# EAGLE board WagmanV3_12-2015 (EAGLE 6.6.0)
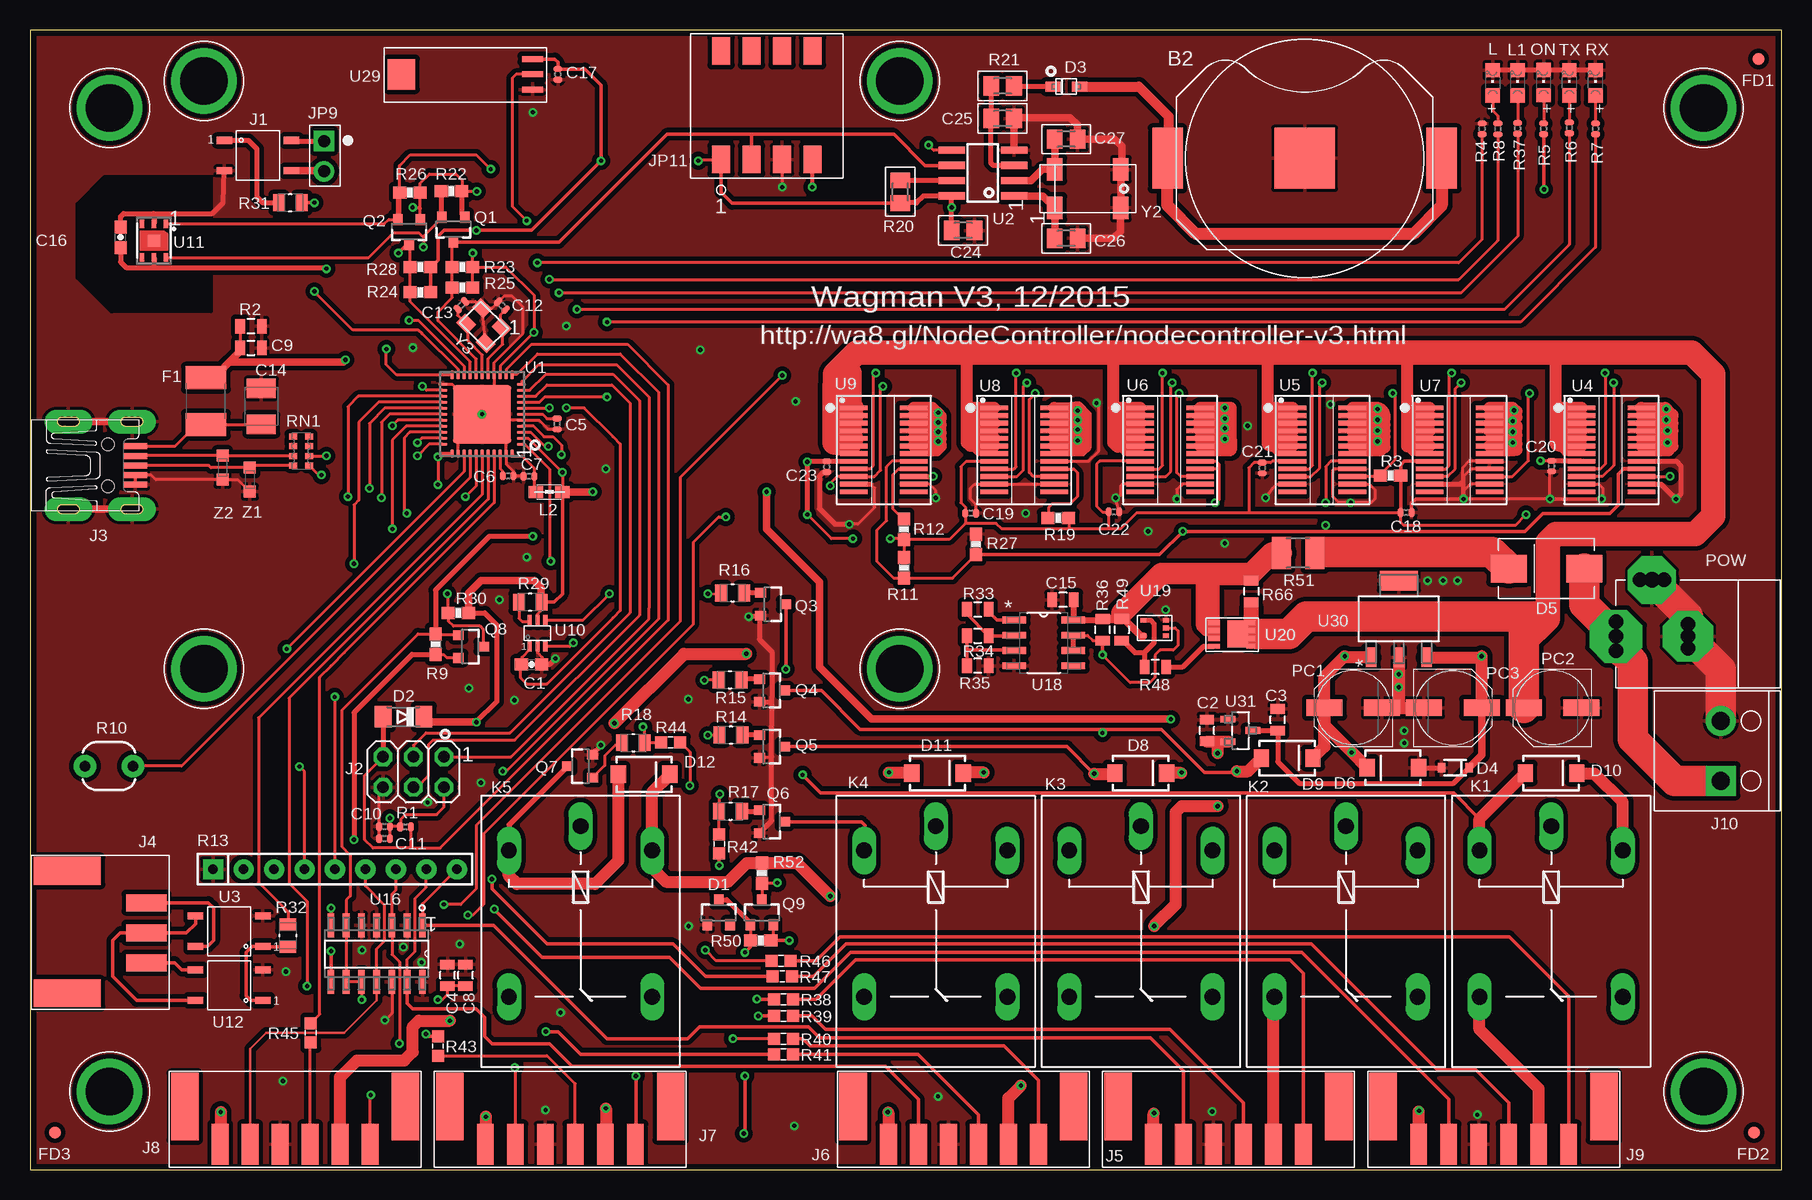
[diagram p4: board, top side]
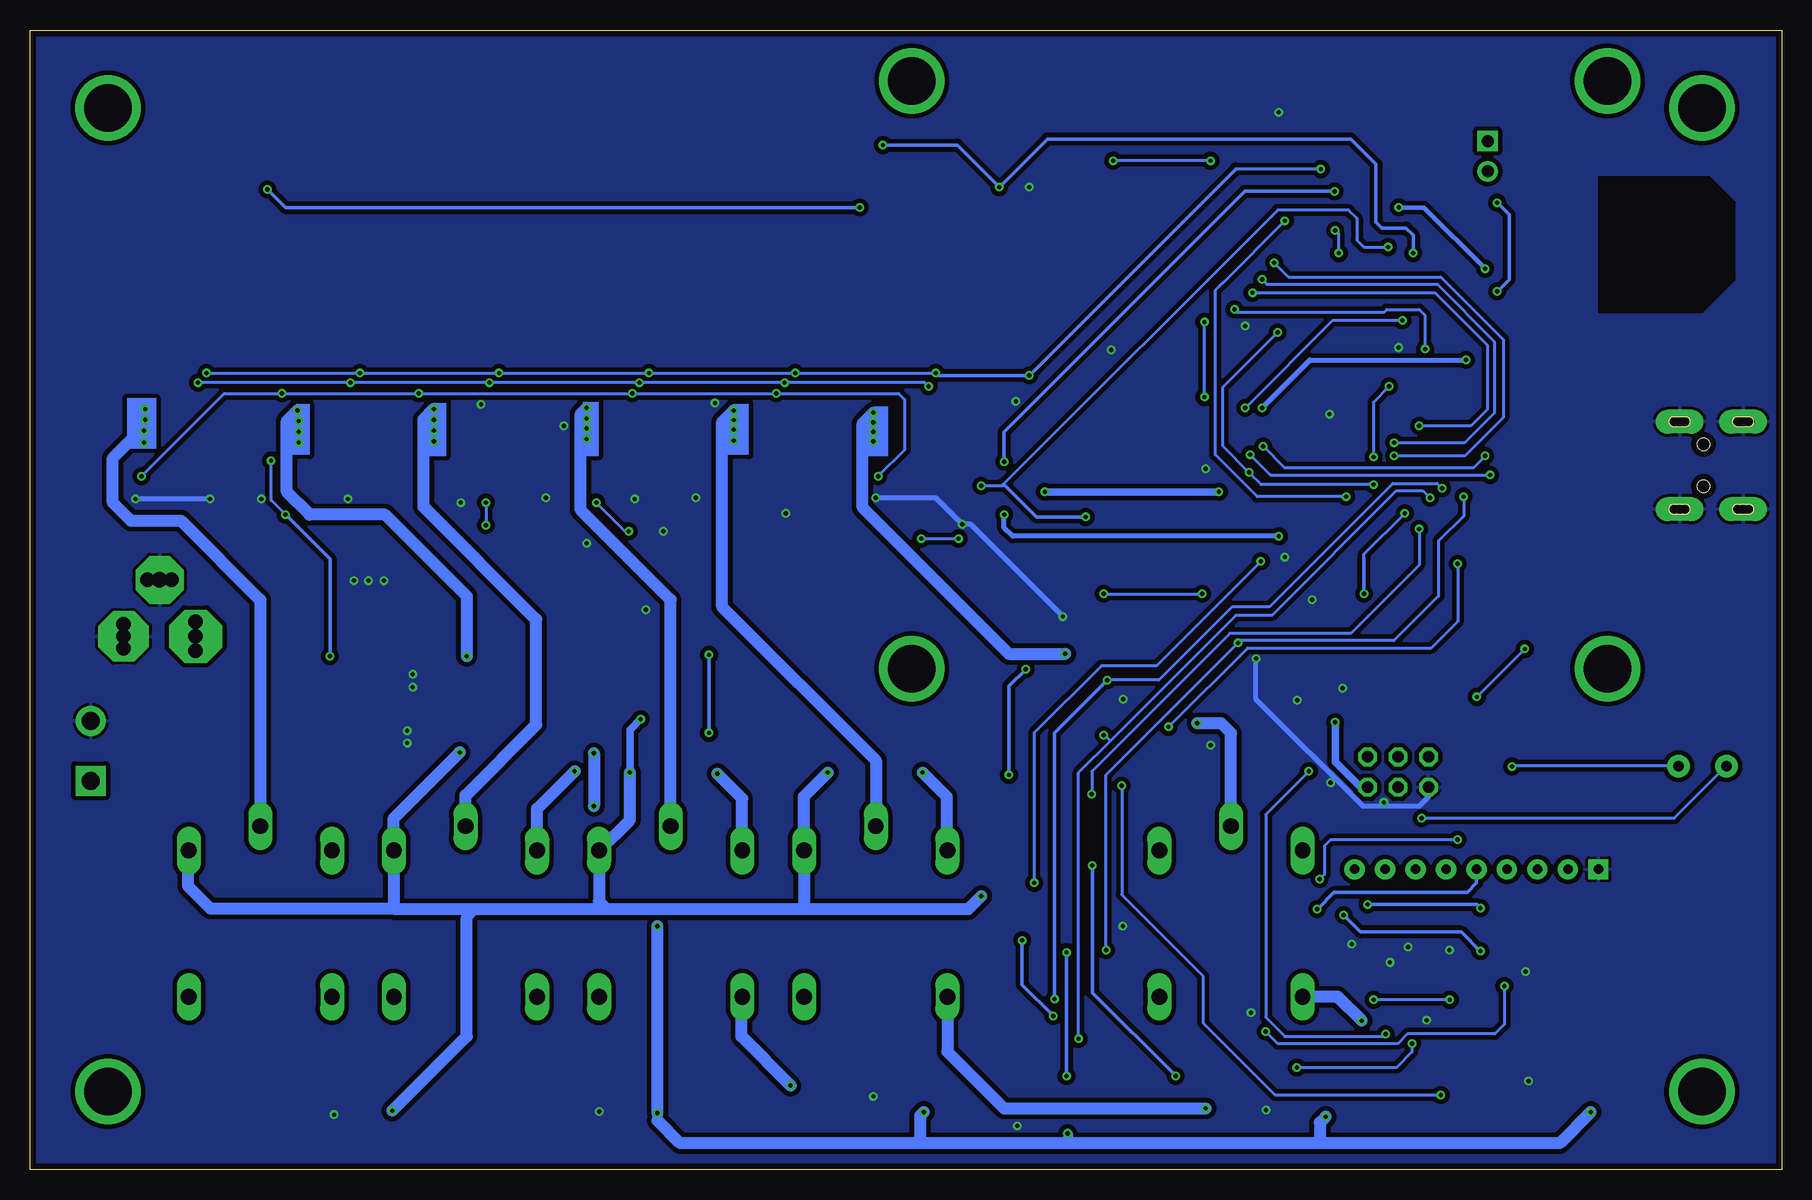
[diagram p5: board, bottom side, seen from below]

Size 146 x 95 mm. Coordinates in mm from the lower left corner, seen from the top.
Outline: 146,95 0,95 0,0 146,0 146,95
Copper layers (1*16): Top 0.035mm / dielectric 1.5mm / Bottom 0.035mm
Design rules "default *": minimum track width 10mil, minimum drill 14mil, track to track 15mil, track to pad 15mil, pad to pad 15mil, via to via 15mil, smd to smd 0mil, copper to edge 20mil, drill to drill 10mil, minimum pad ring 5mil, minimum via ring 5mil, stop-mask expansion 2.5mil, vias tented up to drill 10mil, thermal gap 10mil
Net classes: 0 default: width 0.254 mm, drill 0.61 mm, clearance 0.203 mm
tRestrict: area 3.9,71.5 to 15.1,82.8
bRestrict: area 3.9,71.5 to 15.2,82.7

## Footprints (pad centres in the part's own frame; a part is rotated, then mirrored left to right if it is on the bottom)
BAT-HLD-002-SMT = smd 5.08 x 5.08: NEG 0,0 | smd 2.54 x 5.08: POS1 -11.43,0; POS2 11.43,0
0603-CAP = smd 1.1 x 1: 1 -0.85,0; 2 0.85,0
0805 = smd 0.8 x 1.2: 1 -0.9,0; 2 0.9,0
C0402 = smd 0.508 x 0.762: 1 -0.445,0; 2 0.445,0
SMC_B = smd 1.6 x 2.4: + -1.5,0; - 1.5,0
M0805 = smd 1.3 x 1.6: 1 -0.95,0; 2 0.95,0
SOT23-3 = smd 0.8 x 0.9: 1 -0.95,-1; 2 0.95,-1; 3 0,1.1
MINIMELF = smd 1.4 x 1.8: A 1.7,0; C -1.7,0
SOD-323F = smd 1.27 x 0.813: A -1.118,0; K 1.118,0
SOD-323 = smd 0.63 x 0.83: A 1.15,0; C -1.15,0
DO-214AB = smd 3 x 2.3: A 3.15,0; C -3.15,0
SMA-DIODE = smd 1.27 x 1.47: A -2.15,0; C 2.15,0
L1812 = smd 1.9 x 3.4: 1 -1.95,0; 2 1.95,0
FD-1MM = smd 1 x 1: 1 0,0
SOP-4 = smd 1.3 x 0.6: 1 0,0; 2 0,-2.54; 3 5.6,-2.54; 4 5.6,0
2X03 = drill 0.95 pad 1.55 octagon: 1 -2.54,-1.27; 2 -2.54,1.27; 3 0,-1.27; 4 0,1.27; 5 2.54,-1.27; 6 2.54,1.27
UX60-MB-5S8 = smd 2 x 0.5: 1 8.65,1.6; 2 8.65,0.8; 3 8.65,0; 4 8.65,-0.8; 5 8.65,-1.6 | drill 0.8 pad 2 long: M1 3.1,-3.65; M2 3.1,3.65; M3 8.4,3.65; M4 8.4,-3.65 | drill 0.8: P$1 2.57,3.65; P$2 3.62,3.65; P$3 7.895,3.65; P$4 2.595,-3.65; P$5 8.895,3.65; P$6 3.595,-3.65; P$7 7.895,-3.65; P$8 8.895,-3.65 | hole 1.05: 6.4,-1.75; 6.4,1.75
3PIN-PTSM-RA-2.5MM = smd 1.4 x 3.4: 1 -2.44,0; 2 0.06,0; 3 2.56,0 | smd 2.3 x 5.6: M1 -5.1,-6.6; M2 5.1,-6.6
6PIN-PTSM-2.5MM = smd 1.4 x 3.4: 1 -6.25,0; 2 -3.75,0; 3 -1.25,0; 4 1.25,0; 5 3.75,0; 6 6.25,0 | smd 2.3 x 5.6: M1 -9.2,-3.15; M2 9.2,-3.15
TB2-5MM = drill 1.5 pad 2.5 square: 1 -2.5,0 | drill 1.5 pad 2.5: 2 2.5,0
CONN_2PIN_P2.54MM = drill 1 pad 1.676 square: 1 0,0 | drill 1 pad 1.676: 2 2.54,0
147721-3 = smd 1.52 x 2.29: 1 0,0; 2 2.54,0; 3 5.08,0; 4 7.62,0; P$5 7.62,9.04; P$6 5.08,9.04; P$7 2.54,9.04; P$8 0,9.04
G5LE = drill 1.321 long: 1 -7.493,-5.969; 2 -7.493,5.969; O 4.699,5.969; P -9.525,0; S 4.699,-5.969
CHIPLED_0805 = smd 1.2 x 1.2: A 0,-1.05; C 0,1.05
0805' = smd 1.2 x 1: 1 -1.1,0; 2 1.1,0
MH3.964 = drill 3.962 pad 5.461: 1 0,0
PANASONIC_D = smd 3 x 1.4: + 2.4,0; - -2.4,0
POWERSUPPLY_DC-21MM = drill 1.2 pad 4.4 octagon: 1 0,-6 | drill 1.2 pad 4.2 octagon: 2 0,0 | drill 1.3 pad 4 octagon: 3 -4.7,-3 | drill 1.2: 4 -4.7,-4; 5 -4.7,-2; 6 -1,0; 7 1,0; 8 -1.2,-6; 9 1.2,-6
R0402 = smd 0.508 x 0.762: 1 -0.445,0; 2 0.445,0
0603-RES = smd 1.1 x 1: 1 -0.85,0; 2 0.85,0
PHOTOCELL-KIT = drill 0.9 pad 1.88: 1 -2,0; 2 2,0
RPACK-SIP-PTH-8-LP = drill 0.8 pad 1.676 square: P$1 0,0 | drill 0.8 pad 1.676: P$2 0,-2.54; P$3 0,-5.08; P$4 0,-7.62; P$5 0,-10.16; P$6 0,-12.7; P$7 0,-15.24; P$8 0,-17.78; P$9 0,-20.32
RESC2013X65N = smd 1.016 x 1.397: 1 -0.94,0; 2 0.94,0
PTC-0603 = smd 1 x 1: 1 -0.8,0; 2 0.8,0
R1210 = smd 1.6 x 2.7: 1 -1.4,0; 2 1.4,0
CAY16 = smd 0.5 x 0.65: 1 -1.2,-0.675; 2 -0.4,-0.675; 3 0.4,-0.675; 4 1.2,-0.675; 5 1.2,0.675; 6 0.4,0.675; 7 -0.4,0.675; 8 -1.2,0.675
QFN44ML7X7 = smd 0.75 x 0.275: 1 -3.275,2.5; 2 -3.275,2; 3 -3.275,1.5; 4 -3.275,1; 5 -3.275,0.5; 6 -3.275,0; 7 -3.275,-0.5; 8 -3.275,-1; 9 -3.275,-1.5; 10 -3.275,-2; 11 -3.275,-2.5; 23 3.275,-2.5; 24 3.275,-2; 25 3.275,-1.5; 26 3.275,-1; 27 3.275,-0.5; 28 3.275,0; 29 3.275,0.5; 30 3.275,1; 31 3.275,1.5; 32 3.275,2; 33 3.275,2.5 | smd 0.275 x 0.75: 12 -2.5,-3.275; 13 -2,-3.275; 14 -1.5,-3.275; 15 -1,-3.275; 16 -0.5,-3.275; 17 0,-3.275; 18 0.5,-3.275; 19 1,-3.275; 20 1.5,-3.275; 21 2,-3.275; 22 2.5,-3.275; 34 2.5,3.275; 35 2,3.275; 36 1.5,3.275; 37 1,3.275; 38 0.5,3.275; 39 0,3.275; 40 -0.5,3.275; 41 -1,3.275; 42 -1.5,3.275; 43 -2,3.275; 44 -2.5,3.275 | smd 4.826 x 4.826: EXP 0,0
SO08 = smd 0.6 x 2.2: 1 -1.905,-2.6; 2 -0.635,-2.6; 3 0.635,-2.6; 4 1.905,-2.6; 5 1.905,2.6; 6 0.635,2.6; 7 -0.635,2.6; 8 -1.905,2.6
QSOP24 = smd 0.4 x 2.3: 1 -3.493,-2.5; 2 -2.857,-2.5; 3 -2.223,-2.5; 4 -1.587,-2.5; 5 -0.953,-2.5; 6 -0.318,-2.5; 7 0.318,-2.5; 8 0.953,-2.5; 9 1.587,-2.5; 10 2.223,-2.5; 11 2.857,-2.5; 12 3.493,-2.5; 13 3.493,2.5; 14 2.857,2.5; 15 2.223,2.5; 16 1.587,2.5; 17 0.953,2.5; 18 0.318,2.5; 19 -0.318,2.5; 20 -0.953,2.5; 21 -1.587,2.5; 22 -2.223,2.5; 23 -2.857,2.5; 24 -3.493,2.5
SOT-363 = smd 0.35 x 0.85: 1 -0.65,-1.1; 2 0,-1.1; 3 0.65,-1.1; 4 0.65,1.1; 5 0,1.1; 6 -0.65,1.1
DD8-3X3MM = smd 0.4 x 0.7: 1 -1,-1.4; 2 0,-1.4; 3 1,-1.4; 4 1,1.4; 5 0,1.4; 6 -1,1.4 | smd 1 x 1: EXP 0,0
SOIC127P600X175-14N = smd 1.981 x 0.559: 1 -2.362,3.81; 2 -2.362,2.54; 3 -2.362,1.27; 4 -2.362,0; 5 -2.362,-1.27; 6 -2.362,-2.54; 7 -2.362,-3.81; 8 2.362,-3.81; 9 2.362,-2.54; 10 2.362,-1.27; 11 2.362,0; 12 2.362,1.27; 13 2.362,2.54; 14 2.362,3.81
SOIC127P600X175-8N = smd 1.981 x 0.559: 1 -2.464,1.905; 2 -2.464,0.635; 3 -2.464,-0.635; 4 -2.464,-1.905; 5 2.464,-1.905; 6 2.464,-0.635; 7 2.464,0.635; 8 2.464,1.905
SOT-353 = smd 0.5 x 0.4: 1 0,0; 2 0,-0.65; 3 0,-1.3; 4 1.9,-1.3; 5 1.9,0
SIS413 = smd 0.99 x 0.405: 1 0,0; 2 0,-0.66; 3 0,-1.32; 4 0,-1.98 | smd 0.76 x 0.405: 5 3.075,-1.98; 6 3.075,-1.32; 7 3.075,-0.66; 8 3.075,0 | smd 1.725 x 2.235: PAD 1.992,-0.96
HIH4030 = smd 0.51 x 1.78: 1 -1.27,0; 2 0,0; 3 1.27,0 | smd 2.54 x 2.29: 4 0,10.925
SOT230P700X180-4N = smd 1.626 x 0.889: 1 -3.2,2.311; 2 -3.2,0; 3 -3.2,-2.311 | smd 1.626 x 3.175: 4 3.2,0
SOT95P237X112-3N = smd 0.559 x 1.27: 1 -0.94,-1.041; 2 0.94,-1.041; 3 0,1.041
CRYSTAL-CITIZEN-CM2XXC = smd 1.3 x 1.9: P$1 -2.75,-1.6; P$2 2.75,-1.6; P$3 2.75,1.6; P$4 -2.75,1.6
CRYSTAL-3.2-2.5 = smd 1.3 x 1.05: 1 -1.15,-0.925; 2 1.15,-0.925; 3 1.15,0.925; 4 -1.15,0.925
CT/CN0603 = smd 1 x 1: 1 -1,0; 2 1,0

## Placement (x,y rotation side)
B2  CR2016  [BAT-HLD-002-SMT]  106.25,84.3 180 top
C1  100nF  [0603-CAP]  41.8,42.1 0 top
C2  1uF  [0805]  98.1,36.6 90 top
C3  1uF  [0805]  104,37.5 90 top
C4  0.1uF  [0805]  34.8,16.2 90 top
C5  1uF  [C0402]  43.94,62.16 270 top
C6  100n  [C0402]  39.86,57.82 0 top
C7  1uF  [C0402]  41.59,57.79 180 top
C8  10uF  [0805]  36.3,16.2 90 top
C9  100n  [0805]  18.42,68.5 0 top
C10  100n  [C0402]  29.55,28.59 180 top
C11  100n  [C0402]  29.55,27.59 180 top
C12  22pF  [C0402]  39.35,72.02 315 top
C13  22pF  [C0402]  35.96,72.06 225 top
C14  22u  [SMC_B]  19.28,63.62 90 top
C15  1uF  [0805]  86.1,47.5 180 top
C16  100nF  [0603-CAP]  7.55,77.71 90 top
C17  100n  [C0402]  44,91.3 270 top
C18  0.1uF  [C0402]  114.71,54.77 0 top
C19  0.1uF  [C0402]  78.41,54.72 0 top
C20  0.1uF  [C0402]  126.82,58.64 270 top
C21  0.1uF  [C0402]  102.72,58.49 270 top
C22  0.1uF  [C0402]  90.36,54.82 0 top
C23  0.1uF  [C0402]  66.42,58.59 270 top
C24  100nF  [M0805]  77.78,78.29 0 top
C25  100pF  [M0805]  81.07,87.62 0 top
C26  10pF  [M0805]  86.38,77.63 0 top
C27  8.2pF  [M0805]  86.38,85.9 0 top
D1  BZX84C2V4LT1GOSCT-ND  [SOT23-3]  57.4,21.4 0 top
D2  CD1206-S01575  [MINIMELF]  31.13,37.75 180 top
D3  PMEG6002EJ  [SOD-323F]  86.38,90.28 180 top
D4  MM3Z3V6T1GOSCT-ND  [SOD-323]  118.8,33.5 180 top
D5  SK810L-TPMSCT-ND  [DO-214AB]  126.4,50.1 0 top
D6  SMAZ5V6-FDICT-ND  [SMA-DIODE]  113.6,33.5 180 top
D8  [SMA-DIODE]  92.59,33.05 0 top
D9  [SMA-DIODE]  104.79,34.3 0 top
D10  [SMA-DIODE]  126.79,33.05 0 top
D11  [SMA-DIODE]  75.64,33.05 0 top
D12  [SMA-DIODE]  51.19,32.95 0 top
DRILEGEND  [DRILEGEND]  not placed on the board
F1  MF-MSMF050-2 500mA  [L1812]  14.67,64.06 90 top
FD1  FIDUCIAL-1MM  [FD-1MM]  144.1,92.6 180 top
FD2  FIDUCIAL-1MM  [FD-1MM]  143.7,3.1 180 top
FD3  FIDUCIAL-1MM  [FD-1MM]  2.1,3.1 180 top
J1  CPC1125N  [SOP-4]  16.2,85.8 0 top
J2  3x2M  [2X03]  31.97,33.13 180 top
J3  MINI-USB-UX60-MB-5S8  [UX60-MB-5S8]  0.1,58.7 0 top
J4  PXC_277-2066-1-ND  [3PIN-PTSM-RA-2.5MM]  9.7,19.8 270 top
J5  PXC-277-2076-1-ND  [6PIN-PTSM-2.5MM]  99.9,2.1 180 top
J6  PXC-277-2076-1-ND  [6PIN-PTSM-2.5MM]  77.8,2.1 180 top
J7  PXC-277-2076-1-ND  [6PIN-PTSM-2.5MM]  44.2,2.1 180 top
J8  PXC-277-2076-1-ND  [6PIN-PTSM-2.5MM]  22.1,2.1 180 top
J9  PXC-277-2076-1-ND  [6PIN-PTSM-2.5MM]  122,2.1 180 top
J10  277-2518-ND  [TB2-5MM]  140.95,34.9 90 top
JP9  [CONN_2PIN_P2.54MM]  24.5,85.75 270 top
JP11  147721-3  [147721-3]  57.6,84.2 0 top
K1  G5LE  [G5LE]  126.8,19.1 270 top
K2  G5LE  [G5LE]  109.7,19.1 270 top
K3  G5LE  [G5LE]  92.6,19.1 270 top
K4  G5LE  [G5LE]  75.5,19.1 270 top
K5  G5LE  [G5LE]  45.89,19.1 270 top
L  green  [CHIPLED_0805]  121.93,90.6 0 top
L1  green  [CHIPLED_0805]  124,90.6 0 top
L2  MH2029-300Y  [0805']  43.28,56.5 180 top
MH1  MH-3.964  [MH3.964]  139.5,88.5 180 top
MH2  MH-3.964  [MH3.964]  139.5,6.51 180 top
MH3  MH-3.964  [MH3.964]  6.64,88.5 180 top
MH4  MH-3.964  [MH3.964]  6.64,6.51 180 top
MH5  MH-3.964  [MH3.964]  72.5,41.75 180 top
MH6  MH-3.964  [MH3.964]  14.5,41.75 180 top
MH7  MH-3.964  [MH3.964]  14.5,90.75 180 top
MH8  MH-3.964  [MH3.964]  72.5,90.75 180 top
ON  blue  [CHIPLED_0805]  126.17,90.61 0 top
PC1  4.7uF  [PANASONIC_D]  110.3,38.5 180 top
PC2  47u  [PANASONIC_D]  126.9,38.5 180 top
PC3  1uF  [PANASONIC_D]  118.6,38.5 0 top
POW  POWERSUPPLY_DC21MMX  [POWERSUPPLY_DC-21MM]  138.2,44.45 270 top
Q1  BSS138  [SOT23-3]  35.29,78.4 180 top
Q2  BSS138  [SOT23-3]  31.6,78.2 180 top
Q3  MMBT2222A  [SOT23-3]  61.9,47.12 270 top
Q4  MMBT2222A  [SOT23-3]  61.8,39.94 270 top
Q5  MMBT2222A  [SOT23-3]  61.8,35.26 270 top
Q6  MMBT2222A  [SOT23-3]  61.8,29 270 top
Q7  MMBT2222A  [SOT23-3]  45.9,33.62 90 top
Q8  BSS138  [SOT23-3]  36.7,43.6 270 top
Q9  BSS138  [SOT23-3]  61,21.4 0 top
R1  10K  [R0402]  31.3,28.56 0 top
R2  10K  [0805]  18.42,70.3 180 top
R3  22K  [0603-RES]  113.4,57.85 180 top
R4  10K  [R0402]  121.03,86.76 90 top
R5  1K  [R0402]  126.16,86.76 90 top
R6  1K  [R0402]  128.31,86.84 90 top
R7  1K  [R0402]  130.49,86.76 90 top
R8  1K  [R0402]  122.35,86.75 90 top
R9  10K  [0603-RES]  33.8,43.8 270 top
R10  PHOTOCELLPTH-KIT  [PHOTOCELL-KIT]  6.59,33.63 0 top
R11  43K  [0603-RES]  72.85,50.16 270 top
R12  10K  [0603-RES]  72.85,53.38 90 top
R13  23K  [RPACK-SIP-PTH-8-LP]  15.26,25.03 90 top
R14  1K  [RESC2013X65N]  58.43,36.22 180 top
R15  1K  [RESC2013X65N]  58.35,40.82 180 top
R16  1K  [RESC2013X65N]  58.57,48.07 180 top
R17  1K  [RESC2013X65N]  58.39,29.87 180 top
R18  1K  [RESC2013X65N]  50.29,35.58 0 top
R19  10K  [0603-RES]  85.71,54.31 180 top
R20  10K  [M0805]  72.54,81.51 270 top
R21  1K  [M0805]  81.07,90.34 0 top
R22  10K  [0603-RES]  35.14,81.55 180 top
R23  10K  [0603-RES]  36.04,75.24 180 top
R24  4.7K  [0603-RES]  32.54,73.13 0 top
R25  4.7K  [0603-RES]  36.04,73.53 0 top
R26  10K  [0603-RES]  31.68,81.45 180 top
R27  54K  [0603-RES]  78.85,52.11 90 top
R28  10K  [0603-RES]  32.54,75.24 180 top
R29  1K  [RESC2013X65N]  41.7,47.3 0 top
R30  10K  [0603-RES]  35.7,46.4 180 top
R31  150R  [RESC2013X65N]  21.7,80.6 0 top
R32  150R  [RESC2013X65N]  21.5,19.5 90 top
R33  34K7  [0805]  79,46.7 0 top
R34  6K25  [0805]  79,44.5 0 top
R35  37K2  [0805]  79,42 180 top
R36  4.7k  [0805]  89.4,45 90 top
R37  1K  [R0402]  124,86.8 90 top
R38  PRG18BB470MB1RB  [PTC-0603]  62.8,14.2 180 top
R39  PRG18BB470MB1RB  [PTC-0603]  62.8,12.8 180 top
R40  PRG18BB470MB1RB  [PTC-0603]  62.8,10.9 180 top
R41  PRG18BB470MB1RB  [PTC-0603]  62.8,9.6 180 top
R42  PRG18BB470MB1RB  [PTC-0603]  57.45,27.15 90 top
R43  PRG18BB470MB1RB  [PTC-0603]  34,10.3 90 top
R44  PRG18BB470MB1RB  [PTC-0603]  53.4,35.6 180 top
R45  PRG18BB470MB1RB  [PTC-0603]  23.4,11.4 90 top
R46  PRG18BB470MB1RB  [PTC-0603]  62.6,17.4 180 top
R47  PRG18BB470MB1RB  [PTC-0603]  62.7,16.1 180 top
R48  220R  [0805]  93.8,41.9 180 top
R49  1K  [0805]  91,45 270 top
R50  10K  [0603-RES]  60.9,19.1 0 top
R51  BLE32P  [R1210]  105.7,51.4 180 top
R52  10K  [0603-RES]  61,24.7 270 top
R66  0R  [0805]  101.8,48.2 270 top
RN1  22R  [CAY16]  22.6,59.9 90 top
RX  yellow  [CHIPLED_0805]  130.49,90.6 0 top
TX  yellow  [CHIPLED_0805]  128.31,90.6 0 top
U1  ATMEGA32U4-XUMU  [QFN44ML7X7]  37.69,62.96 180 top
U2  MCP79412  [SO08]  79.43,83.07 90 top
U3  CPC1125N  [SOP-4]  19.4,18.6 180 top
U4  ACS764-QSOP24  [QSOP24]  131.82,60 270 top
U5  ACS764-QSOP24  [QSOP24]  107.73,60 270 top
U6  ACS764-QSOP24  [QSOP24]  95.04,60 270 top
U7  ACS764-QSOP24  [QSOP24]  119.15,60 270 top
U8  ACS764-QSOP24  [QSOP24]  82.86,60 270 top
U9  ACS764-QSOP24  [QSOP24]  71.17,60 270 top
U10  SN74LVC1G175DCKR  [SOT-363]  42.3,44.7 0 top
U11  HTU21D  [DD8-3X3MM]  10.34,77.44 180 top
U12  CPC1017N  [SOP-4]  19.4,14.1 180 top
U16  MCP3428-E/SL  [SOIC127P600X175-14N]  28.9,18 270 top
U18  TMP01FSZ  [SOIC127P600X175-8N]  84.5,43.9 0 top
U19  NL17SZ14D  [SOT-353]  94.7,44.5 180 top
U20  SIS413DN  [SIS413]  98.7,45.6 0 top
U29  HIH4030  [HIH4030]  41.9,91.3 90 top
U30  MCP1825S-3302E/DB  [SOT230P700X180-4N]  114.1,45.9 90 top
U31  MCP1700T-1802E/TT  [SOT95P237X112-3N]  100.9,36.6 270 top
Y2  32.768 kHz  [CRYSTAL-CITIZEN-CM2XXC]  88.18,81.77 0 top
Y3  16MHz KX-7  [CRYSTAL-3.2-2.5]  37.83,70.35 135 top
Z1  CG0603MLC-05E  [CT/CN0603]  18.33,57.52 270 top
Z2  CG0603MLC-05E  [CT/CN0603]  16.06,58.52 270 top

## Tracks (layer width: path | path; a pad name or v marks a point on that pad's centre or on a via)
1V8  (via drill 0.36 pad 0.71)
  Top 0.254: Q9.1 R50.1
  Top 0.305: R50.1 60.05,18.55 v59.6,18.1 | v59.6,7.8 59.6,3.1 v59.5,3
  Top 0.406: D1.3 58.1,22.5 60.05,20.55 Q9.1
  Top 0.61: 98.14,35.66 C2.1 | J7.6 38,2.15
  Top 0.813: 93.65,4.65 v93.7,4.7 | v71.5,4.8 71.55,4.75 | 15.9,2.15 J8.6
  Top 1.016: J5.6 93.65,4.65 | 71.55,4.75 J6.6 | v15.9,4.8 15.9,2.15 | U31.2 99,35.66 | 99,35.66 98.14,35.66 | v99,34.7 99,35.66 | v99,30.3 96,30.3 95.5,29.8 95.5,22.1 v93.7,20.3 | 38,2.15 v38,4.4
  Bottom 0.305: v59.6,18.1 v59.6,7.8
  Bottom 0.813: 93.7,4.1 v93.7,4.7 | v59.5,3 59.5,2.2
  Bottom 1.016: v93.7,4.7 v93.7,20.3 | v99,34.7 v99,30.3 | v15.9,4.8 18.5,2.2 38.5,2.2 | 38.5,2.2 59.5,2.2 71.8,2.2 | 71.8,2.2 91.8,2.2 93.7,4.1 | v71.5,4.8 71.8,4.5 71.8,2.2 | v38,4.4 38.5,3.9 38.5,2.2
1V8D7  (via drill 0.36 pad 0.71)
  Top 0.254: Q9.2 61.95,19.3 R50.2
  Top 0.305: R50.2 v63.3,19.1 | v60.7,12.8 R39.2
  Bottom 0.305: v63.3,19.1 63.3,15.4 v60.7,12.8
3V3  (via drill 0.36 pad 0.71)
  Top 0.254: Q2.1 32.53,79.22 32.53,80.1 | 35.99,79.65 Q1.1 | Q8.1 33.8,44.55 R9.1 32.35,44.65 26,38.3 26,26.9 26.7,26.2 26.7,22.8 26.36,22.46 U16.6 U16.9 U16.10 27.63,14.15 v27.65,14.15 | 10.34,75.44 10.34,75.26 10.4,75.2 | C8.1 C4.1 34.8,14.6 34.35,14.15 v34,14.15 | v37.25,81.55 R22.1 36,82.5 35.5,83 33.3,83 32.53,82.23 R26.1 32.53,80.1 | v31.9,80.2 32.43,80.2 arc-90 32.53,80.1 | v124.7,54.6 123.8,53.7 114.5,53.7 114.27,53.93 C18.1 101.6,54.77 | R12.1 R11.1 | v125.9,59.1 125.92,59.08 C20.1 | U5.8 103.55,59.05 103.43,58.93 C21.1 102.03,58.93 101.6,58.5 101.6,54.77 | 80.35,59.03 78.03,59.03 77.6,58.6 77.6,55.6 77.97,55.23 C19.1 77.97,53.87 | 77.97,53.87 76.63,52.53 R12.1 | R12.1 72.78,52.6 v71.7,52.6 | v68.6,52.6 66.8,52.6 v64.8,54.6 | 101.6,54.77 92.27,54.77 90.9,53.4 89.9,53.4 | U6.8 89.15,59.05 88.9,58.8 88.9,55.3 89.38,54.82 C22.1 89.9,54.8 89.9,53.4 | 89.9,53.4 86.6,53.4 | 86.6,53.4 81,53.4 80.53,53.87 77.97,53.87 | R19.1 86.6,54.27 86.6,53.4
  Top 0.305: C18.1 114.25,54.77 R3.1 114.25,58.75 114.55,59.05 U7.8
  Top 0.406: R22.1 35.99,79.65 | U4.8 126.86,59.05 C20.1 126.81,59.1 | U9.8 68.66,59.03 C23.1 64.83,59.03 v64.8,59 v64.8,54.6 | U8.8 80.35,59.03 | v41.9,52.8 38.3,52.8 33.8,48.3 R9.1 | C16.1 7.55,75.65 8,75.2 10.4,75.2 24.6,75.2 v24.7,75.1 | U11.5 10.34,75.44 | 32.4,81.32 R26.1 | D4.C 118.65,32.2 105.8,32.2 104,34 C3.1 U31.3
  Top 0.61: PC3.+ 121,34.55 D4.C
  Top 1.016: v121,42.8 | PC3.+ v121,42.8 | U30.3 120.9,42.7 v121,42.8
  Bottom 0.254: v27.65,14.15 v34,14.15 | v124.7,54.6 125.9,55.8 v125.9,59.1 | v71.7,52.6 v68.6,52.6
  Bottom 0.305: v64.8,59 64.8,61.5 44.75,81.55 v37.25,81.55 | v121,42.8 121,50.9 v124.7,54.6
  Bottom 0.356: v24.7,75.1 29.8,80.2 v31.9,80.2
  Bottom 0.406: v41.9,52.8 64.1,52.8 64.8,53.5 v64.8,54.6
3V3D5*  (via drill 0.36 pad 0.71)
  Top 0.254: Q8.2 34.75,42.65 34.5,42.9 33.85,42.9 R9.2
  Top 0.305: R47.2 56.3,16.1 53.6,18.8 43.1,18.8 38.5,23.4 v38.5,24.2
  Top 0.406: v27,27.5 27,38.1 31.85,42.95 R9.2
  Bottom 0.254: v27,27.5 37.6,27.5 38.1,27 38.1,24.6 v38.5,24.2
5IN
  Top 0.254: 101.8,49.7 R66.1
  Top 0.305: C15.1 86.96,47.46 | 89.31,45.8 arc90 R36.2
  Top 0.4: U20.3 98.7,44.3 98.8,44.3 99,44.5 99,45.3 U20.1
  Top 0.5: 86.96,47.46 U18.8 89.31,45.8
  Top 0.61: U19.5 92.6,44.5 91.2,45.9 R49.1
  Top 0.7: R36.2 R49.1
  Top 0.813: 91,46.4 R49.1 | R66.1 98.9,49.1
  Top 1: U20.2 98.06,44.94 97.7,45.3 97.7,49 98.2,49.5 | 98.2,49.5 98.4,49.7 | U20.1 98.7,49 98.2,49.5
  Top 1.778: R51.2 103.5,51.4 101.8,49.7 98.4,49.7 94.3,49.7 91,46.4
+5V  (via drill 0.36 pad 0.71)
  Top 0.254: 44.3,56.58 L2.1 | R23.1 R25.2 36.96,73.3 | 44.2,56.68 L2.1 | R29.2 42.64,46.64 42.3,46.3 U10.5 | C10.1 30.83,28.59 R1.1 30.9,28.61 30.9,29.2 31.3,29.6 33.9,29.6 34.51,30.21 J2.2 34.51,30.91 | C10.1 C11.1 | v55.7,84.1 55.8,84.2 JP11.1 | U1.2 41.54,60.96 v44.38,58.12 L2.1 | C10.1 v30,29.3 | R23.1 39.66,75.24 42,72.9 v42,69.8 39.19,66.99 U1.14 | U1.34 34.28,59.69 v34,59.4 v34,57.1 | U1.24 33.04,64.96 v32.7,65.3 | R23.1 v36.89,76.39 v36.9,76.4 | 123.69,61.59 v123.6,61.5 | 123.65,60.95 123.6,60.9 v123.6,60.6
  Top 0.305: R20.2 58.54,80.56 57.6,81.5 JP11.1 | U29.3 43.73,92.57 44,92.3 C17.1 46.26,91.75 47.6,90.4 v47.6,84.1 41.8,78.3 v37.2,78.3 34.5,78.3 34,77.8 34,75.8 33.44,75.24 R28.1 R24.2 | L2.1 44.38,47.98 43.7,47.3 R29.2 | R5.1 126.2,86.28 v126.2,81.7
  Top 0.406: C24.1 v76.83,80.2 U2.8 74.47,81.17 73.9,80.6 72.58,80.6 R20.2 | 42.74,47.2 R29.2 | R30.1 37.9,46.4 38.9,45.4 38.9,39 v37.2,37.3 | 123.9,60 123.58,59.68 U7.18 123.72,59.68 | U7.24 | 123.72,60.32 123.9,60.5 | U7.20 123.65,60.95 123.9,61.2 | 123.69,61.59 123.9,61.8 | 123.72,62.22 v123.6,62.4 | 123.74,62.86 123.9,62.7 | 77.84,33.1 D11.C | v96,33.1 95.95,33.05 | 51.9,26.55 K5.2 | v109.6,42.8
  Top 0.61: R29.2 42.6,47.34 42.6,48.5 42,49.1 37.6,49.1 36.55,48.05 R30.1 | v37.2,37.3 32.78,37.3 D2.C | v46.9,56.5 L2.1 | v95.1,37.55 70.15,37.55 65.8,41.9 65.8,49 61.4,53.4 v61.4,56.5 | 128.99,33 D10.C
  Top 0.813: 115.75,4.85 v115.8,4.9
  Top 1.016: PC1.+ 107.9,37.05 v110.17,34.77 D6.C | 123.9,60 123.9,60.5 123.9,61.2 123.9,61.8 123.9,62 v123.6,62.4 123.9,62.7 123.9,63.2 123.85,63.25 | 123.85,63.25 123.6,63.5 U7.24 | U7.19 123.72,60.32 | U7.21 123.69,61.59 | U7.22 123.72,62.22 | U7.23 123.74,62.86 | J9.6 115.75,4.85 | v66.7,22.8 63.95,25.55 R52.1 59.75,25.55 58.2,24 53,24 51.9,25.1 51.9,26.55 | v79.5,33.1 77.84,33.1 | K1.2 132.77,30.63 130.4,33 128.99,33 | PC1.+ 107.9,41.1 v109.6,42.8 109.7,42.7 U30.1 | 95.95,33.05 D8.C | D9.C 107.9,35.26 PC1.+ | K5.2 51.86,31.47 D12.C | v123.7,63.3 123.85,63.25
  Bottom 0.254: v47.6,84.1 v55.7,84.1 | v30,29.3 8.92,29.3 R10.1 | v42,69.8 46.6,65.2 46.6,60.34 v44.38,58.12 43.36,57.1 v34,57.1 | v34,59.4 34,64 v32.7,65.3 | v36.9,76.4 36.9,78 v37.2,78.3
  Bottom 0.305: v126.2,81.7 124.7,80.2 v76.83,80.2
  Bottom 0.406: 110.4,35 arc-90 v110.17,34.77
  Bottom 0.61: v37.2,37.3 37.2,34 35.06,31.86 J2.2 | v46.9,56.5 v61.4,56.5 | v95.1,37.55 96,36.65 v96,33.1
  Bottom 0.813: 109.6,21 108.9,21.7
  Bottom 1.016: K4.2 81.5,26.62 | 81.2,21.7 67.8,21.7 v66.7,22.8 | 81.2,21.7 97.9,21.7 | 97.9,21.7 108.9,21.7 115.6,21.7 115.67,21.77 | 115.67,21.77 K2.2 115.67,29.28 v110.17,34.77 | 81.5,26.62 81.5,22 81.2,21.7 | K1.2 132.8,26.56 132.8,23.6 130.97,21.77 115.67,21.77 | 97.9,21.7 98.57,22.37 K3.2 96,29.16 v96,33.1 | 81.5,26.62 81.5,31.1 v79.5,33.1 | v109.6,42.8 109.6,47.8 116.4,54.6 122.7,54.6 124.6,56.5 124.6,62.4 v123.7,63.3 | 109.6,21 109.6,11.1 v115.8,4.9
A0  (via drill 0.36 pad 0.71)
  Top 0.254: U1.36 36.19,58.19 v21.4,43.4 | R13.P$5 25.42,39.38 v25.4,39.4
  Top 0.305: J9.5 118.25,5.85 106,18.1 68.4,18.1 65.4,15.1 55.9,15.1 53.3,17.7 42.7,17.7 39.45,20.95 v38.7,21.7
  Bottom 0.254: v25.4,39.4 v21.4,43.4
  Bottom 0.305: R13.P$5 25.42,23.88 26.2,23.1 37.3,23.1 v38.7,21.7
A1  (via drill 0.36 pad 0.71)
  Top 0.254: U1.37 36.69,57.69 12.63,33.63 R10.2 | R13.P$4 22.88,33.17 v22.45,33.6
  Bottom 0.254: R10.2 22.42,33.63 v22.45,33.6
A2  (via drill 0.36 pad 0.71)
  Top 0.254: U1.38 37.19,56.99 v36.3,56.1 | U29.2 40.5,91.3 40.2,91 40.2,80.3 v41.4,79.1
  Bottom 0.254: v36.3,56.1 43.7,56.1 47.2,59.6 47.2,73.3 46.8,73.7 46.5,74 v41.4,79.1
A3
  Top 0.254: U1.39 37.69,56.29 19.05,37.65 19.05,23.95 21.5,21.5 R32.2
A4  (via drill 0.36 pad 0.71)
  Top 0.254: U1.40 38.19,55.89 21.6,39.3 21.6,23.85 23.1,22.35 v23.1,15.3
  Top 0.305: R41.2 45.9,9.6 44,11.5 v43,11.5
  Bottom 0.254: v43,11.5 42,10.5 32,10.5 31.2,11.3 23.9,11.3 23.1,12.1 23.1,15.2
  Bottom 0.305: 23.1,15.2 v23.1,15.3
A5
  Top 0.254: U1.41 38.69,55.59 26.2,43.1 25.1,42 24.15,41.05 24.15,12.95 R45.2
ADD_V5  (via drill 0.36 pad 0.71)
  Top 0.254: U9.17 71.85,59.05 71.4,58.6 71.4,54.1 70.6,53.3 70.6,50.7 71.99,49.31 R11.2 76.9,49.31 R27.1 | U5.17 108.45,59.05 108,58.6 v108,55.6 | U6.17 98.85,59.05 99,58.9 | 99,58.9 99,58.5 98.91,58.41 U6.16 | 99,58.9 99.1,58.8 99.1,55.8 98.9,55.6 v98.8,55.6 | v108,53.7 108,53.2
  Top 0.305: U6.17 | U5.17 110.21,59.03 | U4.16 134.31,58.4 | 132.8,58.4 132.4,58 132.4,55.4 131.7,54.7 126.1,54.7 124.6,53.2 108,53.2 v96.1,53.2 94.16,51.26 R27.1
  Top 0.35: 134.31,58.4 132.8,58.4
  Top 0.406: U6.17 97.52,59.03
  Bottom 0.254: v108,55.6 v108,53.7 | v98.8,55.6 96.4,53.2 v96.1,53.2
AREF
  Top 0.254: U1.42 39.2,58.44 39.42,58.22 C6.1
AVCC
  Top 0.254: U1.44 40.27,59.5 41,59.5 42.03,58.47 C7.1 42.03,56.65 L2.2
BAT
  Top 0.813: D3.A 92.42,90.28 94.9,87.8 94.9,83.4 94.8,83.3
  Top 1.016: B2.POS1 117.68,80.38 115.3,78 97.2,78 94.8,80.4 94.8,83.3 94.8,84.28 B2.POS2
D0/RX  (via drill 0.36 pad 0.71)
  Top 0.254: U10.1 41.65,43.35 41,42.7 41,42.15 C1.1 40.9,42.05 40.9,41 41.4,40.5 43.1,40.5 48.6,46 49.2,46.6 49.2,54.4 49.2,60.5 48.6,61.1 46.2,63.5 v44.7,63.5 | U1.20 36.18,66.99 32.37,70.8 v31.6,70.8
  Bottom 0.254: v44.7,63.5 37.4,70.8 v31.6,70.8
D1/TX  (via drill 0.36 pad 0.71)
  Top 0.254: U1.21 35.68,66.71 32.67,69.67 32.34,70 26.9,70 v23.7,73.2
  Top 0.305: R31.2 v23.7,80.6
  Bottom 0.305: v23.7,73.2 22.7,74.2 22.7,79.6 v23.7,80.6
D2/SDA  (via drill 0.36 pad 0.71)
  Top 0.254: U1.19 36.69,67.35 31.7,72.34 31.7,73.22 | 31.7,73.22 R24.1 | 31.7,73.22 R28.2 | R28.2 31.69,77.01 Q2.3 | U2.5 75.33,84.97 v74.9,85.4 | 31.63,75.3 R28.2 | v65.2,81.9 65.2,84.18 JP11.4 65.22,81.92 v65.2,81.9
  Top 0.305: v30.7,76.4 31.4,77.1 Q2.3
  Bottom 0.305: v74.9,85.4 68.7,85.4 v65.2,81.9 61.2,85.9 35.9,85.9 33.8,83.8 33.8,79 33.3,78.5 31.3,78.5 30.7,77.9 v30.7,76.4
D3/SCL
  Top 0.254: U1.18 37.19,67.57 34,70.76 34,71.5 35.2,72.7 35.2,73.22 R25.1 R23.2 35.19,77.2 Q1.3
  Top 0.305: 60,86.3 72,86.3 74.6,83.7 U2.6 | 60,86.3 53.1,86.3 44.1,77.3 Q1.3 | 60,86.3 60.14,86.16 JP11.2
D4*  (via drill 0.36 pad 0.71)
  Top 0.254: U1.25 27.36,64.46 26.5,63.6 v26.5,56.1 | v45.3,43.9 45,43.6 U10.3 | R46.2 57.2,17.4 v56.3,18.3
  Bottom 0.254: v26.5,56.1 26.5,54.5 28.6,52.4 28.6,47.8 32.3,44.1 45.1,44.1 v45.3,43.9 56.3,32.9 v56.3,18.3
D5*  (via drill 0.36 pad 0.71)
  Top 0.254: U1.31 31.66,61.46 31.2,61 31.2,54.9 v31.4,54.7 | v34.8,48 34.8,46.45 R30.2 34.9,46.35 34.9,45.7 35.3,45.3 37.5,45.3 37.8,45 Q8.3
  Bottom 0.254: 34.8,51 34.8,51.3 v31.4,54.7
  Bottom 0.305: v34.8,48 34.8,51
D6*  (via drill 0.36 pad 0.71)
  Top 0.254: U1.27 29.56,63.46 28.3,62.2 v28.3,56.8 | R15.2 57.39,40.8 v56.2,40.8
  Top 0.305: R38.2 v60.6,14.2
  Bottom 0.254: v56.2,40.8 51.9,40.8 45.8,46.9 42.7,46.9 32.4,57.2 28.7,57.2 v28.3,56.8 28.5,57
  Bottom 0.305: v60.6,14.2 60.6,36.4 v56.2,40.8
D7  (via drill 0.36 pad 0.71)
  Top 0.254: U1.1 41.24,60.46 43.3,58.4 43.3,50.8 v43.4,50.7 | Q9.3 R52.2 62.25,23.85 v62.3,23.9
  Bottom 0.254: v43.4,50.7 52.1,42 56.7,42 62.3,36.4 v62.3,23.9
D_N
  Top 0.254: RN1.7 16.08,59.5 Z2.1 8.77,59.52 J3.2
D_P
  Top 0.254: RN1.8 18.51,58.7 Z1.1 15.08,58.52 14.9,58.7 J3.3
FAULT_PU  (via drill 0.36 pad 0.71)
  Top 0.254: U8.15 83.62,57.78 83.3,58.1 83.3,64.2 v83.8,64.7 | U6.15 95.92,57.78 95.6,58.1 95.6,64.5 v95.8,64.7 | U7.15 123.58,57.78 124.9,59.1 124.9,64.6 v125,64.7 | v113.6,64.7 113.8,64.5 113.8,59.2 112.38,57.78 U5.15 | U4.15 136.68,57.78 v136.7,57.8
  Top 0.305: 112.38,57.78 112.48,57.78 R3.2
  Top 0.406: U9.15 75.18,57.78 v75.3,57.8
  Bottom 0.254: v136.7,57.8 129.8,64.7 v125,64.7 v113.6,64.7 v95.8,64.7 v83.8,64.7 73.6,64.7 73.1,64.2 73.1,60 v75.3,57.8
GND  (via drill 0.36 pad 0.71)
  Top 0.254: 39.59,62.46 U1.5 42.44,62.46 43.18,61.72 C5.2 | 39.59,62.46 39.09,62.96 38.9,62.96 | 38.9,62.96 U1.EXP | 39.59,62.46 39.69,62.36 U1.43 39.7,59.67 39.7,58.8 40.3,58.2 C6.2 | 38.9,62.96 38.69,63.17 U1.15 38.69,67.29 41.1,69.7 41.1,71.9 40.2,72.8 39.5,72.8 C12.1 38.52,71.82 Y3.2 | U1.23 35.19,65.46 35.9,64.75 | 35.9,64.75 U1.EXP | U1.35 35.69,60.96 U1.EXP | U10.2 42.3,43.1 42.7,42.7 42.7,42.15 C1.2 | C11.2 C10.2 | C10.2 29.03,28.67 | C10.2 29.11,31.54 J2.6 | U4.11 130.76,57.14 131.1,56.8 131.1,56 v131,55.9 | 126.82,58.12 C20.2 126.7,58.2 v126.7,55.9 v119.5,55.9 | U7.14 120.04,57.14 119.55,56.65 | 119.55,56.65 119.5,56.6 v119.5,55.9 | U7.16 120.11,58.41 119.5,57.8 119.5,56.7 119.55,56.65 | U7.17 119.95,59.05 119.4,58.5 119.4,57.3 119.4,56 v119.5,55.9 | U5.16 110.22,58.4 108.7,58.4 108.6,58.3 108.6,56.1 109.1,55.6 v110.1,55.6 111.8,55.6 112.1,55.9 112.1,56.7 111.66,57.14 U5.14 | U5.11 105.19,57.1 103.9,57.1 103.6,56.8 v103,56 | U9.11 69.86,57.14 | 70.08,57.14 70.4,56.82 70.4,55.2 69,53.8 v68.3,53.8 | 40.2,57.83 C6.2 | C7.2 41.12,57.82 C6.2 | v75.5,56 75.5,56.6 74.96,57.14 U9.14 | Q5.2 60.89,34.4 61.83,34.4 | 35.9,64.75 v37.68,62.98 | J3.5 J3.4 10.1,57.9 10.48,57.52 Z2.2 17.33,57.52 Z1.2 | U16.12 30.17,13.03 v29.59,12.45 | JP11.3 62.68,81.92 v62.7,81.9 | C13.1 37.11,72.37 Y3.2 | Y3.4 Y3.2 | U6.11 91.04,57.14 90.9,57 90.9,56.2 v90.5,56 90.5,55.8 C22.2 | U6.14 96.04,57.14 95.6,56.7 v95.6,55.9 | U8.14 U8.11 78.74,57.14 78.4,56.8 78.4,55.9 78.86,55.45 C19.2 | U8.17 88.25,59.05 89.1,59.9 89.1,63.7 v88.9,63.9
  Top 0.305: 126.8,58.12 126.7,58.12 | 126.82,58.12 126.8,58.12 | 126.8,58.12 126.8,58.1 | v131,55.9 v126.7,55.9 | v119.5,55.9 115.5,55.9 115.15,55.55 C18.2
  Top 0.406: U2.4 C25.2 | C16.2 7.55,79.45 7.8,79.7 10.3,79.7 | U11.2 10.34,79.66 10.3,79.7 | 10.3,79.7 15.2,79.7 16.1,80.6 J1.2 | U4.14 135.96,57.14 v137.2,55.9 137.6,56.3 137.6,58.7 137.25,59.05 U4.17 | U7.11 119.24,57.14 119.4,57.3 | C23.2 66.14,58.15 65.8,57.8 65.8,55.1 67.1,53.8 v68.3,53.8 | 69.86,57.14 70.08,57.14 | v43.8,42.6 43.3,42.1 C1.2 | 61.82,39 61.82,39.38 61.83,39.39 61.83,43.17 60.8,44.2 60.8,46.17 Q3.2 60.83,46.1 v59.9,46.1 | 61.82,39 61.82,37.03 61.83,37.03 61.83,34.4 61.83,29.08 Q6.2 | Q4.2 61.82,39 | Q7.2 46.9,34.68 v47.59,35.37 | RX.C TX.C ON.C L1.C L.C | D6.A D4.A 117.7,33.5
  Top 0.61: C26.2 90.33,77.63 90.9,78.2 90.9,80.14 Y2.P$2 Y2.P$3 91,83.44 91,85.3 90.4,85.9 C27.2 87.3,85.93 87.3,87.1 86.7,87.7 82,87.7 82.03,87.67 U2.4 | J3.M1 J3.M4 | J3.M2 J3.M3
  Top 1.016: PC1.- 114.1,38.5 | 114.1,38.5 PC3.- | U30.2 114.1,38.5
  Top 2.54: J10.2 140.95,41.7 POW.2 138.2,46.15 POW.3
  Bottom 0.406: v75.5,56 70.5,56 v68.3,53.8 | v131,55.9 v137.2,55.9 | 67.8,53.8 v68.3,53.8 | v59.9,46.1 67.6,53.8 v68.3,53.8 | J2.6 29.43,31.07 30.2,30.3 34.9,30.3 43.8,39.2 v43.8,42.6
  other vias: 41.91,88.14 55.88,68.33 63.82,64.05 48.01,58.42 36.58,40.13 40.39,39.12 37.59,32.26 33.15,30.61 35.81,18.8 21.34,16.51 21.08,7.37 114.55,36.58 114.55,35.56 120.65,4.57 98.55,4.83 75.69,6.1 63.71,3.64 42.97,4.95 44.23,13.08 27.69,18.29 31.11,18.54 32.64,17.27 94.66,46.67 41.4,51.05 39.12,47.5 31.91,68.52 44.71,70.32 119,49.1 116.5,49.1 117.8,49.1 114.1,41.3 114.1,40.2 99.6,52.2 54.89,39.22 93.2,53.2 83,54.7 54.9,20.3 101.5,62 108.4,63.8
  pour Bottom: 0,0 146,0 146,95 0,95
  pour Top: 0,0 146,0 146,95 0,95
HWB  (via drill 0.36 pad 0.71)
  Top 0.254: R4.1 121.03,77.53 119.1,75.6 v42.3,75.6 | U1.33 33.26,60.46 v32.3,59.5
  Bottom 0.254: v32.3,59.5 26.4,59.5 23.2,62.7 23.2,69.2 28.4,74.4 41.1,74.4 v42.3,75.6
IO8  (via drill 0.36 pad 0.71)
  Top 0.254: U1.28 29.96,62.96 29.3,62.3 v29.3,56 | R40.2 v58.6,10.9 | R14.2 57.47,36.2 v56.5,36.2
  Bottom 0.254: 55.95,35.75 45.5,46.2 42.5,46.2 32.1,56.6 29.9,56.6 v29.3,56 29.5,56.2 | 55.95,35.75 58.6,33.1 v58.6,10.9 | v56.5,36.2 56.4,36.2 55.95,35.75
IO9*  (via drill 0.36 pad 0.71)
  Top 0.254: R37.1 124,77.8 119.3,73.1 v44.1,73.1 | U1.29 30.66,62.46 v30.2,62
  Bottom 0.254: v44.1,73.1 28.9,73.1 24.5,68.7 24.5,63.4 25.9,62 v30.2,62
IO10*  (via drill 0.36 pad 0.71)
  Top 0.254: R17.2 57.65,29.9 | U1.30 31.36,61.96 30.2,60.8 v30.2,53.4 | v57.5,31.3 57.45,31.25 R17.2 | R42.2 | R42.2 R17.2
  Bottom 0.254: v30.2,53.4 30.2,50.4 35.9,44.7 46,44.7 57.5,33.2 v57.5,31.3
IO11*  (via drill 0.36 pad 0.71)
  Top 0.254: U1.12 40.19,66.29 40.2,66.3 40.6,66.3 42.3,68 49.2,68 52.4,64.8 52.4,45.9 39.7,33.2 v39.4,33.2
  Top 0.305: R43.2 33.2,11.1 v33,11.3
  Bottom 0.254: v39.4,33.2 43,29.6 43,12.7 41.4,11.1 33.2,11.1 v33,11.3
IO12*  (via drill 0.36 pad 0.71)
  Top 0.254: U1.26 29.06,63.96 27.4,62.3 27.4,55.8 27,55.4 v27,50.5 | R44.2 52.58,35.58 R18.2 51.23,36.77 v51.1,36.9
  Bottom 0.254: v27,50.5 27,45.7 29.2,43.5 44.5,43.5 v51.1,36.9
IO13*  (via drill 0.36 pad 0.71)
  Top 0.254: R8.1 122.35,77.45 119.1,74.2 v43.3,74.2 | U1.32 32.66,60.96 v32.3,60.6
  Bottom 0.254: v32.3,60.6 26.4,60.6 23.9,63.1 23.9,69 28.7,73.8 42.9,73.8 v43.3,74.2
MFP
  Top 0.406: U2.7 72.56,82.44 R20.1
MISO
  Top 0.254: U1.11 41,65.5 41,65.7 42.4,67.1 48.9,67.1 51.6,64.4 51.6,46.8 51.6,45.9 50.2,44.5 40.1,34.4 J2.1
MOSI
  Top 0.254: U1.10 41.66,64.96 43,66.3 48.6,66.3 50.8,64.1 50.8,46.2 40.4,35.8 33.6,35.8 33.2,35.4 33.2,32.8 32.26,31.86 J2.4
N$1
  Top 0.254: 85.35,58.4 87,58.4 87.3,58.1 87.3,56.1 86.7,55.5 85.2,55.5 84.9,55.2 84.9,54.35 R19.2
  Top 0.305: 85.35,58.4 U8.16
N$2
  Top 0.254: RX.A R7.2
N$3
  Top 0.254: ON.A 126.17,87.22 R5.2
N$4
  Top 0.254: TX.A R6.2
N$5
  Top 0.254: U9.16 72.41,58.41 71.9,57.9 71.9,55.1 72.77,54.23 R12.2
N$6
  Top 0.61: J1.3 24.45,83.26 JP9.2
N$7
  Top 0.254: L.A 121.93,88.27 122.35,87.85 R8.2
N$8
  Top 0.305: U18.2 82,44.5 R34.2 78.1,46.3 R33.1
N$9
  Top 0.305: R34.1 78.1,43.3 | 78.1,43.3 R35.2 | U18.3 82,43.3 78.1,43.3
N$10
  Top 0.305: U18.1 80.59,45.8 79.9,46.5 R33.2
N$11  (via drill 0.36 pad 0.71)
  Top 0.305: Q5.3 86.44,35.26 v88.7,33
  Top 0.406: 90.39,33 D8.A
  Top 1.016: v88.7,33 90.39,33
  Bottom 1.016: K3.1 86.63,30.93 v88.7,33
N$12
  Top 0.406: R48.1 96.1,41.9 97.82,43.62 U20.4
N$13
  Top 0.406: U19.4 93.4,45.8 93.7,45.5 93.7,43.9 92.9,43.1 | 92.9,43.1 R48.2 | R49.2 91.1,44.1 92.1,43.1 92.9,43.1
N$14
  Top 0.406: Q5.1 R14.1
N$15
  Top 0.61: U2.2 83.44,82.44 84.4,83.4 85.4,83.4 Y2.P$4 C27.1
N$16  (via drill 0.36 pad 0.71)
  Top 0.254: U18.7 88.17,44.53 88.6,44.1 R36.1 | U19.2 95.45,45.15 95.7,44.9 95.7,43.7 95.3,43.3 94.2,43.3 93.78,42.88 93.78,41.04 93.34,40.6 91.7,40.6 v89.4,42.9
  Top 0.305: v89.4,42.9 R36.1 | Q4.3 65.96,39.94 69.2,36.7 89.4,36.7 | 89.4,36.7 94.3,36.7 97.9,33.1 100.5,33.1 v100.6,33.2 | v89.4,36.4 89.4,36.7
  Top 0.4: U18.6 U18.7
  Top 1.016: v100.6,33.2 101.54,33.2 D9.A
  Bottom 0.305: v89.4,36.4 v89.4,42.9
  Bottom 1.016: K2.1 103.73,30.07 v100.6,33.2
N$17
  Top 0.61: C26.1 Y2.P$1 84.44,81.17 U2.1
N$18
  Top 0.406: Q4.1 59.36,40.89 R15.1
N$19
  Top 2.54: D5.A 129.55,47.1 POW.1 132.2,43.7 133.6,42.3 133.6,35.9 137.1,32.4 J10.1
N$20  (via drill 0.36 pad 0.71)
  Top 0.305: Q3.3 v63,41.7 | 120.83,29.24 118.67,31.4 65.9,31.4 v64.4,32.9
  Top 1.016: K1.1 120.83,29.24 D10.A
  Bottom 0.305: v64.4,32.9 64.4,40.3 v63,41.7
N$21
  Top 0.406: D3.K 82.08,90.28 R21.2
N$22
  Top 0.406: Q3.1 R16.1
N$23
  Top 0.406: J1.4 21.85,85.75 JP9.1
N$24  (via drill 0.36 pad 0.71)
  Top 0.305: Q6.3 69.3,29 69.6,28.7 69.6,26.66 K4.1
  Top 0.406: 73.44,33.1 D11.A
  Top 1.016: v71.6,33.1 73.44,33.1
  Bottom 0.406: 69.6,27.1 69.53,27.03 K4.1
  Bottom 1.016: v71.6,33.1 69.6,31.1 69.6,27.1
N$25
  Top 0.254: L1.A R37.2
N$26
  Top 0.406: R17.1 60.72,29.87 Q6.1
N$27
  Top 0.254: R29.1 40.76,45.94 41,45.7 41.6,45.7 U10.6
N$28
  Top 0.406: Q7.3 39.92,28.74 K5.1
  Top 0.813: 39.9,26.57 K5.1
  Top 1.016: D12.A 49.04,25.74 47.1,23.8 40.6,23.8 39.9,24.5 39.9,26.57
N$29
  Top 0.305: J5.1 106.15,16.35 105,17.5 68.8,17.5 65.5,14.2 R38.1
N$30
  Top 0.254: R18.1 48.75,35.35 47.9,34.5 47.9,33.67 Q7.1
N$31
  Top 0.305: J5.3 101.15,5.55 95,11.7 66.3,11.7 65.2,12.8 R39.1
N$32
  Top 0.305: J6.1 84.05,7.45 81.2,10.3 65,10.3 64.4,10.9 R40.1
N$33
  Top 0.305: J6.3 79.05,4.55 74,9.6 R41.1
N$34  (via drill 0.36 pad 0.71)
  Top 0.305: R42.1 v57.45,25.35 | v50.5,7.8 50.5,2.15 J7.1
  Bottom 0.305: v57.45,25.35 57.45,14.75 v50.5,7.8
N$35
  Top 0.254: J7.3 45.45,7.15 43.1,9.5 R43.1
N$36  (via drill 0.36 pad 0.71)
  Top 0.254: J8.1 28.35,6.15 v28.4,6.2 | R44.1 55,34.8 v55,32
  Bottom 0.254: v28.4,6.2 42.2,6.2 48.2,12.2 48.2,16.1 55,22.9 v55,32
N$37
  Top 0.254: J8.3 23.35,10.55 R45.1
N$38
  Top 0.305: J9.1 128.25,14.45 123.3,19.4 67.5,19.4 65.5,17.4 R46.1
N$39
  Top 0.305: J9.3 123.25,5.55 120.5,8.3 117.3,8.3 106.8,18.8 68,18.8 65.3,16.1 R47.1
N$40
  Top 0.406: J1.1 18.2,85.8 18.9,85.1 18.9,81.1 19.4,80.6 R31.1
N$41
  Top 0.305: R32.1 19.44,18.56 U3.1 18.5,18.6 18,18.1 18,14.5 18.4,14.1 U12.1
N$42
  Top 0.305: U3.3 13.8,20.5 13.04,19.74 J4.2 7.54,19.74 6.9,19.1 6.9,16.1 8.9,14.1 U12.4
N$43
  Top 0.305: J4.1 14.86,22.24 15.3,21.8 15.3,19.1 14.8,18.6 U3.4
N$44
  Top 0.305: J4.3 12.06,17.24 12.66,16.64 U12.3
N$45
  Top 1.422: 107.6,51.4 R51.1
  Top 1.93: 107.6,51.5 107.6,51.4
  Top 2.54: D5.C 121.85,51.5 107.6,51.5
NC_POW  (via drill 0.36 pad 0.71)
  Top 0.254: 43,45.7 U10.4 46.1,45.8 v48.3,48 | v56.5,48 57.7,48 R16.2
  Bottom 0.254: v56.5,48 v48.3,48
OP1
  Top 1.016: J9.2 125.75,6.75 120.83,11.67 K1.S
OP2
  Top 0.813: 103.65,14.32 K2.S
  Top 1.016: J5.2 103.65,14.32
OP3  (via drill 0.36 pad 0.71)
  Top 1.016: J6.2 81.55,5.95 v82.6,7
  Bottom 0.813: 86.7,14.33 K3.S
  Bottom 1.016: 86.7,14.33 86.7,11.1 v82.6,7
OP4  (via drill 0.36 pad 0.71)
  Top 0.813: 48,2.15 J7.2
  Top 1.016: v48,5.1 48,2.15
  Bottom 1.016: K4.S 69.53,9.83 64.8,5.1 v48,5.1
OP5  (via drill 0.36 pad 0.71)
  Top 1.016: J8.2 25.85,7.7 27.25,9.1 31.2,9.1 31.9,9.8 31.9,11.9 32.4,12.4 v35,12.4
  Bottom 1.016: v35,12.4 37,14.4 K5.S
POW1  (via drill 0.36 pad 0.71)
  Top 0.406: U4.18 134.34,59.7 136.7,59.7 136.9,59.9 136.9,60.3 136.88,60.32 | 136.9,62.9 136.8,63 136.66,62.86 | 136.88,62.22 136.9,62.2 136.9,61.6 136.89,61.59 | 136.85,60.95 136.9,60.9
  Top 1.016: U4.24 136.31,63.49 v136.4,63.4 | v136.4,63.4 136.8,63 | 136.9,62.9 136.9,62.8 | v136.4,62.5 136.9,62.2 | U4.23 136.66,62.86 | U4.22 136.88,62.22 | U4.21 135.4,61.59 | 135.4,61.59 136.89,61.59 | U4.20 136.85,60.95 v136.5,60.6 136.78,60.32 | U4.19 136.78,60.32 | 136.9,61.6 v136.4,62.5 | 136.9,62.8 136.3,63.4 | 136.3,63.4 134.4,63.4 134.3,63.5 | v136.5,61.6 135.41,61.6 135.4,61.59 | 136.3,63.4 v136.4,63.4 | 136.9,62.8 v136.4,62.5 | 136.88,60.32 136.78,60.32 | 136.9,60.3 136.9,62.8
  Bottom 1.016: K1.P 126.8,47.5 133.4,54.1 137.6,54.1 139.1,55.6 139.1,59.3 136.8,61.6 v136.5,61.6
POW2  (via drill 0.36 pad 0.71)
  Top 0.254: 112.2,63.5 112.3,63.4 v112.34,63.4 | 112.64,62.86 112.34,62.55 v112.34,62.5 | 112.89,61.59 112.88,61.6 v112.34,61.6 | 112.75,60.95 112.5,60.7 v112.34,60.7
  Top 0.406: 112.9,62.8 112.9,62.6 112.64,62.86 | U5.24 | 112.78,62.22 112.9,62.1 | 112.89,61.59 112.9,61.6 | 112.75,60.95 112.9,61.1 | 112.78,60.32 112.9,60.2 112.9,59.9 112.68,59.68 U5.18
  Top 1.016: 112.9,60.2 112.9,61.1 112.9,61.6 112.9,62.1 112.9,62.6 | U5.24 111.8,63.5 112.2,63.5 arc-90 112.9,62.8 | U5.23 112.64,62.86 | U5.22 112.78,62.22 | U5.21 112.89,61.59 | U5.20 112.75,60.95 | U5.19 112.78,60.32
  Bottom 1.016: K2.P 109.7,31.2 103.8,37.1 103.8,45.86 113.2,55.26 113.2,62.54 v112.34,63.4
POW3  (via drill 0.36 pad 0.71)
  Top 0.254: 99.85,62.55 99.8,62.6 v99.6,62.6 | 99.85,62.22 99.6,61.97 v99.6,61.8 | 100.1,60.95 100.05,60.9 v99.6,60.9 | 100.1,60 arc-90 99.78,59.68 U6.18
  Top 0.406: U6.21 97.55,61.6 | U6.22 99.85,62.22 99.85,62.55 | U6.18 100.1,59.68 | 99.55,62.86 99.55,62.85
  Top 1.016: 98.91,63.49 U6.24 | 97.55,61.6 100.1,61.6 | U6.20 100.1,60.95 | U6.19 100.1,60.32 100.1,60.9 | U6.23 99.55,62.86 99.85,62.56 99.85,62.55 | 99.8,63.5 v99.6,63.5 U6.24 | U6.24 U6.23 | U6.21 U6.23 | 100.1,60.9 100.1,63.49 U6.24 | 100.05,60.9 arc-90 100.1,60.85 100.1,60 arc-90 99.6,60.5 v99.6,60.9 100.1,60.9
  Bottom 1.016: K3.P 92.6,47.5 100.1,55 100.1,63 v99.6,63.5
POW4  (via drill 0.36 pad 0.71)
  Top 0.254: 86.99,63.49 87.2,63.28 v87.34,63.28 | 87.54,62.86 87.34,62.66 v87.34,62.48 | 87.61,61.59 87.52,61.68 v87.34,61.68 | 87.75,60.95 87.58,60.78 v87.34,60.78
  Top 0.406: 87.8,62.7 87.8,62.6 arc90 87.54,62.86 | 86.99,63.49 87,63.5 | 87.72,62.22 87.8,62.3 | 87.61,61.59 87.8,61.4 | 87.75,60.95 87.8,61 | 87.78,60.32 87.8,60.3 87.8,59.82 87.84,59.78 | U8.18 87.78,59.68 88.3,60.2 88.3,63 87.5,63.8 87.11,63.8 86.8,63.49
  Top 1.016: 87.8,60.3 87.8,61 87.8,61.4 87.8,62.3 87.8,62.6 | 87.8,62.7 87,63.5 | U8.24 86.8,63.49 86.99,63.49 | U8.23 87.54,62.86 | U8.22 87.72,62.22 | U8.21 87.61,61.59 | U8.20 87.75,60.95 | U8.19 87.78,60.32
  Bottom 1.016: K4.P 75.5,34.1 88.3,46.9 88.3,62.32 v87.34,63.28
POW5  (via drill 0.36 pad 0.71)
  Top 0.254: 75.84,62.86 75.7,63 v75.7,63.1 | 75.78,62.22 v75.7,62.3 | 75.71,61.59 75.7,61.58 v75.7,61.5 | 75.85,60.95 75.7,60.8 v75.7,60.7
  Top 0.406: 75.9,62.8 75.84,62.86 | U9.24 | 75.78,62.22 75.9,62.1 | 75.71,61.59 75.9,61.4 | 75.85,60.95 75.9,60.9 | 75.82,60.32 75.9,60.4 | U9.18 75.68,59.68 76.2,60.2 76.2,62.6 v75.7,63.1
  Top 1.016: 75.9,60.4 75.9,60.9 75.9,61.4 75.9,62.1 75.9,62.8 | U9.24 75.2,63.5 75.84,62.86 U9.23 | U9.22 75.78,62.22 | U9.21 75.71,61.59 | U9.20 75.85,60.95 | U9.19 75.82,60.32 | v48.7,37.2 54.5,43 v59.7,43
  Bottom 1.016: v59.7,43 64.4,43 76.6,55.2 76.6,62.2 v75.7,63.1 | K5.P 45.89,36.39 46.7,37.2 v48.7,37.2
RD_N  (via drill 0.36 pad 0.71)
  Top 0.254: U1.3 41.74,61.46 42.9,60.3 v43.2,60.3 | RN1.2 v24.7,59.5
  Bottom 0.254: v43.2,60.3 41.4,58.5 25.7,58.5 v24.7,59.5
RD_P  (via drill 0.36 pad 0.71)
  Top 0.254: U1.4 41.98,61.96 42.84,61.1 43.6,61.1 44.3,60.4 v44.3,59.6 | RN1.1 24.07,57.9 v24.3,57.9
  Bottom 0.254: v24.3,57.9 42.6,57.9 v44.3,59.6
RESET
  Top 0.254: U1.13 39.69,66.69 41.8,68.8 49.8,68.8 53.2,65.4 53.2,45.8 34.2,26.8 31.9,26.8 | 31.9,26.8 28.6,26.8 27.9,27.5 27.9,32.87 J2.5 | R1.2 31.74,26.96 31.9,26.8
  Top 0.406: D2.A J2.5
RXLED/SS  (via drill 0.36 pad 0.71)
  Top 0.254: R7.1 130.49,76.89 124.25,70.65 v48.1,70.65 | U1.8 42.46,63.96 42.9,64.4 v48.1,64.4
  Bottom 0.254: v48.1,64.4 v48.1,70.65
SCK
  Top 0.254: U1.9 42.16,64.46 43.1,65.4 48.5,65.4 50,63.9 50,46.4 40,36.4 33,36.4 31.97,35.37 J2.3
SCL_3  (via drill 0.36 pad 0.71)
  Top 0.254: 129.3,57.8 U4.10 131.08,57.78 132,58.7 v132,65.6 | U11.6 28.24,76.04 30.3,78.1 32.4,78.1 32.7,77.8 32.8,77.8 | v66.7,57 66.7,57.2 67.28,57.78 U9.10 70.38,57.78 70.9,58.3 70.9,65.1 v71.1,65.3 | 32.8,77.8 v32.8,76.9 | 34.29,79.45 33.9,78.9 32.8,77.8 | v36.5,21.2 36.9,21.2 37.8,22.1 37.8,28 55.3,45.5 55.3,52.3 57.4,54.4 v58,54.4 | U8.10 82.28,57.78 82.8,58.3 82.8,65.3 v83.1,65.6 | U5.10 106.78,57.78 107.5,58.5 107.5,65.4 v107.7,65.6 | 116.63,57.8 118.2,57.8 118.8,58.4 118.8,65.1 v119.3,65.6 | U6.10 94.68,57.78 95.1,58.2 95.1,65.5 v95.2,65.6
  Top 0.305: 116.63,57.8 U7.10 | v25.1,18.2 U16.8
  Top 0.406: R22.2 34.29,79.45 Q1.2
  Bottom 0.254: 64.8,57 65,57 | 65,57 v66.7,57 | 65,57 64.85,57.15 42,80 36.1,80 35.4,79.3 35.4,77.5 34.8,76.9 v32.8,76.9 | v71.1,65.3 71.4,65.6 v83.1,65.6 v95.2,65.6 95.7,65.6 v107.7,65.6 v119.3,65.6 v132,65.6
  Bottom 0.305: 64.85,57.15 62.1,54.4 v58,54.4 | v25.1,18.2 26.7,19.8 35.1,19.8 v36.5,21.2
SDA_3  (via drill 0.36 pad 0.71)
  Top 0.254: R26.2 30.83,79.38 Q2.2 | Q2.2 30.65,81.25 30.8,81.4 30.8,83.7 31.7,84.6 37.2,84.6 v38.4,83.4 | 68.68,58.4 U9.9 70.01,58.41 70.3,58.7 70.3,66.2 v70.5,66.4 | v131.3,66.4 131.3,58.8 130.9,58.4 129.33,58.4 U4.9 | U11.1 29.54,78.84 29.9,79.2 Q2.2 | 80.37,58.4 82,58.4 82.2,58.6 v82.2,66.4 | v34.5,22.1 35.9,22.1 37.2,23.4 37.2,28.7 54.2,45.7 54.2,57.7 v62.7,66.2 | U5.9 106.61,58.41 106.9,58.7 v106.9,66.4 | U7.9 118.01,58.41 118.3,58.7 118.3,66.2 v118.5,66.4 | U6.9 94.11,58.41 94.4,58.7 v94.4,66.4
  Top 0.305: U8.9 80.37,58.4 | v25.1,21.8 v25.09,21.79 U16.7
  Bottom 0.254: v38.4,83.4 45.5,83.4 | v131.3,66.4 v118.5,66.4 v106.9,66.4 v94.4,66.4 v82.2,66.4 v70.5,66.4
  Bottom 0.305: v34.5,22.1 25.4,22.1 v25.1,21.8 | 45.5,83.4 v62.7,66.2 70.3,66.2 v70.5,66.4
THM0
  Top 0.254: R13.P$9 32.71,22.16 U16.1
  Top 0.305: J5.5 96.15,8.25 93.4,11 65.8,11 64.9,11.9 55.8,11.9 54.8,10.9 48.1,10.9 38.64,20.36 U16.1
THM1
  Top 0.254: U16.13 31.44,17.53 32.1,18.19 32.1,22.6 33.04,23.54 R13.P$8
  Top 0.305: J6.5 74.05,5.85 71.3,8.6 45.2,8.6 43.3,10.5 38.5,10.5 37.9,11.1 37.9,12.7 37.2,13.4 31.9,13.4 31.44,13.86 U16.13 31.4,15.6
THM2  (via drill 0.36 pad 0.71)
  Top 0.254: R13.P$7 30.5,23.3 30.17,22.97 U16.3 30.17,17.93 30.8,17.3 v30.8,10.5 | J7.5 40.45,8.45 v40.4,8.5
  Bottom 0.254: v40.4,8.5 32.1,8.5 30.8,9.8 v30.8,10.5
THM3
  Top 0.203: J8.5 18.35,10.05 19.7,11.4 26.2,11.4 28.9,14.1 U16.11
  Top 0.254: U16.11 28.9,18.4 29.54,19.04 29.54,22.06 27.96,23.64 R13.P$6
TXLED  (via drill 0.36 pad 0.71)
  Top 0.254: R6.1 128.31,77.11 122.9,71.7 v45.6,71.7 | U1.22 30.57,66.23 29.7,67.1 v29.7,68.4
  Bottom 0.254: v29.7,68.4 29.7,71.2 30.2,71.7 32.9,71.7 33.1,71.5 45.4,71.5 v45.6,71.7
UCAP
  Top 0.254: U1.6 42.74,62.96 43.1,62.6 43.34,62.6 C5.1
VBAT
  Top 0.406: R21.1 C25.1 80.1,87.6 80.1,83.9 80.3,83.7 U2.3
VIN_5
  Top 0.305: U9.7 67.22,59.68 66.4,60.5 66.4,61.5 66.9,61 | U9.6 67.38,60.32 67.08,60.62 66.9,60.8 | 66.9,60.9 66.9,61 | 66.9,61 66.9,61.6 67.5,62.2
  Top 0.381: U20.5 U20.6
  Top 0.406: U9.3 68.65,62.2 | U8.7 79.02,59.68 78.38,60.32 | 78.1,67.8 77.8,68.1 | U8.4 78.19,61.59 78.1,61.5 | 78.12,62.22 78.1,62.2 | U8.2 78.16,62.86 78.1,62.8 | 78.1,63.5 78.11,63.49 78.11,68.19 78.1,68.2 | U6.7 91.22,59.68 90.65,60.25 90.72,60.32 | 90.3,68 90.2,68.1 | 90.45,60.95 90.3,61.1 | 90.31,61.59 90.3,61.6 | 90.48,62.22 90.3,62.4 | 90.36,62.86 90.3,62.8 | 90.41,63.49 90.3,63.6 | U5.7 103.92,59.68 103.4,60.2 | 103.4,60.2 103.2,60.4 | 103.2,68 103.1,68.1 | 103.52,60.32 103.4,60.2 | 103.25,60.95 103.2,60.9 | 103.21,61.59 103.2,61.6 | 103.28,62.22 103.2,62.3 | 103.26,62.86 103.2,62.8 | 103.21,63.49 103.2,63.5 | U7.7 115.22,59.68 114.8,60.1 114.8,60.3 114.82,60.32 | 114.8,67.7 114.4,68.1 | U7.5 114.85,60.95 114.8,61 | 114.81,61.59 114.8,61.6 | 114.88,62.22 114.8,62.3 | 114.84,62.86 114.8,62.9 | 114.89,63.49 114.8,63.4 | U4.7 127.92,59.68 127.4,60.2 | 127.4,60.2 127.2,60.4 | 127.2,68 127.3,68.1 | 127.52,60.32 127.4,60.2 | 127.25,60.95 127.2,60.9 | 127.21,61.59 127.2,61.6 | 127.22,62.22 127.2,62.2 | 127.34,62.86 127.2,63 | 127.21,63.49 127.2,63.5 | U20.PAD 101.78,44.64 U20.7 | U9.7
  Top 0.61: U9.3 68.2,61.75 68.5,61.75 U9.4
  Top 0.813: U20.8 U20.7 | U20.7 U20.6 | R66.2 101.8,46.8 101.8,44.97 U20.7
  Top 1.016: 78.1,61 78.1,60.6 78.38,60.32 U8.6 | 78.1,61 78.1,61.5 78.1,62.2 78.1,62.8 78.1,63.5 78.1,67.8 | U8.5 78.15,60.95 78.1,61 | U8.3 78.12,62.22 | U8.1 78.11,63.49 | 90.65,60.25 90.3,60.6 90.3,61.1 90.3,61.6 90.3,62.4 90.3,62.8 90.3,63.6 90.3,68 | U6.6 90.72,60.32 | U6.5 90.45,60.95 | U6.4 90.31,61.59 | U6.3 90.48,62.22 | U6.2 90.36,62.86 | U6.1 90.41,63.49 | 103.2,60.4 103.2,60.9 103.2,61.6 103.2,62.3 103.2,62.8 103.2,63.5 103.2,68 | U5.6 103.52,60.32 | U5.5 103.25,60.95 | U5.4 103.21,61.59 | U5.3 103.28,62.22 | U5.2 103.26,62.86 | U5.1 103.21,63.49 | 114.8,60.3 114.8,61 114.8,61.6 114.8,62.3 114.8,62.9 114.8,63.4 114.8,67.7 | U7.6 114.82,60.32 | U7.4 114.81,61.59 | U7.3 114.88,62.22 | U7.2 114.84,62.86 | U7.1 114.89,63.49 | 127.2,60.4 127.2,60.9 127.2,61.6 127.2,62.2 127.2,63 127.2,63.5 127.2,68 | U4.6 127.52,60.32 | U4.5 127.25,60.95 | U4.4 127.21,61.59 | U4.3 127.22,62.22 | U4.2 127.34,62.86 | U4.1 127.21,63.49 | 124.4,43.8 124.4,46 124.5,46.1
  Top 1.27: 102.25,44.65 101.8,45.1 101.8,46.8 | U9.5 U9.6 | U9.2 U9.3 U9.4 U9.5 | U9.5 68.25,60.95 68.2,60.9 | 66.9,60.8 66.9,60.9 67,61 | 67,61.6 67,61 | 67,61 67.1,61 | 67,61 66.9,61 67,60.9
  Top 1.676: U9.2 68.5,63.03 68.5,66.4 68.2,66.1 68.2,63.1 68.59,63.49 U9.1
  Top 2.032: 126.5,46.9 124.5,44.9 | 126.5,46.9 126.5,45.9 124.4,43.8 | 126.5,46.9 126.5,52.3 127.2,53 138.8,53 140.3,54.5 140.3,66.3 138.5,68.1 127.3,68.1 114.4,68.1 103.1,68.1 90.2,68.1 77.8,68.1 68.9,68.1 67.1,66.3 67.1,65.4 67.08,65.38 67.08,60.62
  Top 2.54: 125.4,46.1 124.5,46.1 106.4,46.1 104.95,44.65 102.25,44.65 | PC2.+ 124.5,44.9 | 67.5,61.2 67.8,60.9 68.2,60.9
VUSB  (via drill 0.36 pad 0.71)
  Top 0.254: U1.7 43.16,63.46 arc90 v43.3,63.5 | R2.2 C9.1 17.52,68.22 | 15.75,66.45 15.31,66.01 F1.2
  Top 0.406: 16.8,67.5 16.6,67.3
  Top 0.61: 17.52,68.22 16.6,67.3 | 16.6,67.3 15.75,66.45 | v26.3,67.5 26.1,67.3 16.6,67.3
  Bottom 0.406: v26.3,67.5 39.3,67.5 v43.3,63.5
VUSBD
  Top 0.254: J3.1 12.1,60.3 13.6,61.8 14.36,61.8 F1.1 C14.+
XTAL1
  Top 0.254: U1.17 37.69,67.91 36.5,69.1 36.5,70.37 Y3.3 35.65,71.23 C13.2
XTAL2
  Top 0.254: U1.16 38.19,67.59 39.4,68.8 39.4,70.09 Y3.1 | 38.99,70.41 Y3.1 | C12.2 39.2,71.24 39.2,70.29 Y3.1
(copper drawn outside any net)
  shapes: Bottom area x11

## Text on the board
tPlace: + | + | + | + | 1 | 1 | 1 | 1 | Wagman V3, 12/2015 | 1 | http://wa8.gl/NodeController/nodecontroller-v3.html | 1 | 1
DrillLegend: LAYER-STACK
DrillLegend_01-16: 01-16
DrillLegend_01-20: 01-20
